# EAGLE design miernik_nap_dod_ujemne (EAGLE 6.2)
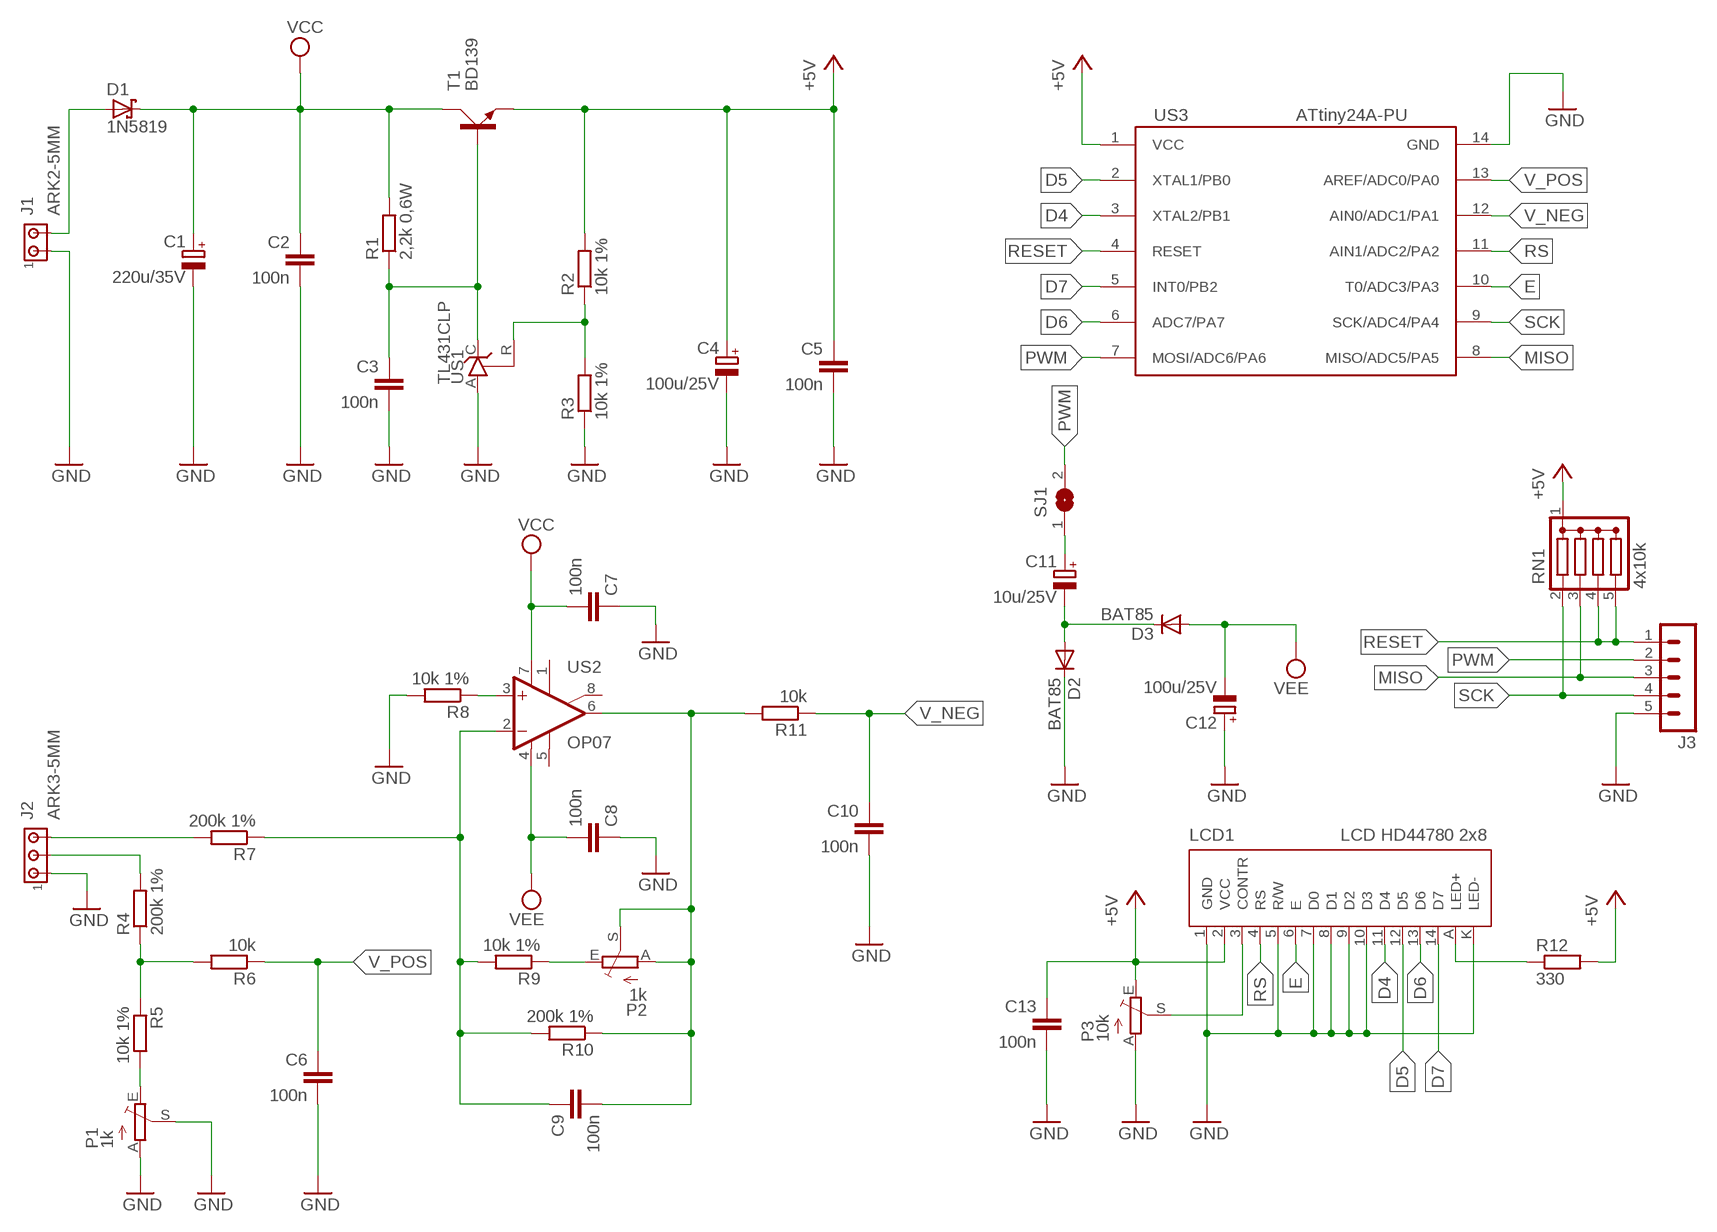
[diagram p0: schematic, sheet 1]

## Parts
C1  220u/35V  CPOL-EUTT5D9L  [TT5D9L]
C2  100n  C-EU050-025X075  [C050-025X075]
C3  100n  C-EU050-030X075  [C050-030X075]
C4  100u/25V  CPOL-EUTT2D6L  [TT2D6L]
C5  100n  C-EU050-025X075  [C050-025X075]
C6  100n  C-EU050-025X075  [C050-025X075]
C7  100n  C-EU050-025X075  [C050-025X075]
C8  100n  C-EU050-025X075  [C050-025X075]
C9  100n  C-EU050-025X075  [C050-025X075]
C10  100n  C-EU050-025X075  [C050-025X075]
C11  10u/25V  CPOL-EUTT2D6L  [TT2D6L]
C12  100u/25V  CPOL-EUTT2D6L  [TT2D6L]
C13  100n  C-EU050-025X075  [C050-025X075]
D1  1N5819  SCHOTTKY-DIODEF126Z12  [F126Z12]
D2  BAT85  BAT81  [DO34-7]
D3  BAT85  BAT81  [DO34-7]
J1  ARK2-5MM  [2PIN-5MM]
J2  ARK3-5MM  [3PIN-5MM]
J3  MA05-1  [MA05-1]
LCD1  LCD HD44780 2x8  LCD_ZLACZE-MINI  [LCD_HD44780_1X6_NAD-ELEMENTAMI_Z-PODSW]
P1  1k  TRIM_EU-B64Y  [B64Y]
P2  1k  TRIM_EU-B64Y  [B64Y]
P3  10k  TRIM_EU-CA6V  [CA6V]
R1  2,2k 0,6W  R-EU_0207/7  [0207/7]
R2  10k 1%  R-EU_0207/7  [0207/7]
R3  10k 1%  R-EU_0207/7  [0207/7]
R4  200k 1%  R-EU_0207/7  [0207/7]
R5  10k 1%  R-EU_0207/7  [0207/7]
R6  10k  R-EU_0207/7  [0207/7]
R7  200k 1%  R-EU_0207/7  [0207/7]
R8  10k 1%  R-EU_0207/7  [0207/7]
R9  10k 1%  R-EU_0207/7  [0207/7]
R10  200k 1%  R-EU_0207/7  [0207/7]
R11  10k  R-EU_0207/7  [0207/7]
R12  330  R-EU_0207/7  [0207/7]
RN1  4x10k  DRAB_REZ_1X4  [RN-5]
SJ1  SJ  [SJ]
T1  BD139  [TO126AV]
US1  TL431CLP  [TO92-CLP]
US2  OP07  OP07N  [DIL08]
US3  ATtiny24A-PU  ATTINY24/44/84-PU  [DIL14]

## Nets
+5V: C4.+ C5.1 C13.1 LCD1.2(VCC) P3.E R2.2 R12.2 RN1.1(C) T1.E US3.1(VCC)
D4: LCD1.11(D4) US3.3(XTAL2/PB1)
D5: LCD1.12(D5) US3.2(XTAL1/PB0)
D6: LCD1.13(D6) US3.6(ADC7/PA7)
D7: LCD1.14(D7) US3.5(INT0/PB2)
E: LCD1.6(E) US3.10(T0/ADC3/PA3)
GND: C1.- C2.2 C3.2 C4.- C5.2 C6.2 C7.1 C8.1 C10.2 C12.+ C13.2 D2.C J1.P$1 J2.P$1 J3.5 LCD1.1(GND) LCD1.5(R/W) LCD1.7(D0) LCD1.8(D1) LCD1.9(D2) LCD1.10(D3) LCD1.K(LED-) P1.A P1.S P3.A R3.1 R8.2 US1.A US3.14(GND)
MISO: J3.3 RN1.3 US3.8(MISO/ADC5/PA5)
N$1: LCD1.3(CONTR) P3.S
N$2: C11.- D2.A D3.C
N$3: C11.+ SJ1.1
N$4: J2.P$2 R4.2
N$5: LCD1.A(LED+) R12.1
N$6: P1.E R5.2
N$7: R4.1 R5.1 R6.2
N$8: D1.A J1.P$2
N$9: R8.1 US2.3(+IN)
N$10: C9.2 P2.A P2.S R10.1 R11.2 US2.6(OUT)
N$11: C3.1 R1.1 T1.B US1.C
N$12: P2.E R9.1
N$14: C9.1 R7.1 R9.2 R10.2 US2.2(-IN)
N$15: J2.P$3 R7.2
N$33: R2.1 R3.2 US1.R
PWM: J3.2 SJ1.2 US3.7(MOSI/ADC6/PA6)
RESET: J3.1 RN1.4 RN1.5 US3.4(RESET)
RS: LCD1.4(RS) US3.11(AIN1/ADC2/PA2)
SCK: J3.4 RN1.2 US3.9(SCK/ADC4/PA4)
V_NEG: C10.1 R11.1 US3.12(AIN0/ADC1/PA1)
V_POS: C6.1 R6.1 US3.13(AREF/ADC0/PA0)
VCC: C1.+ C2.1 C7.2 D1.C R1.2 T1.C US2.7(V+)
VEE: C8.2 C12.- D3.A US2.4(V-)
Unconnected: US2.1(ON1) US2.5(OPT) US2.8(ON2)

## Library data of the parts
C1 C4 C11 C12 = rcl:CPOL-EU: POLARIZED CAPACITOR, European symbol
C2 C3 C5-C10 C13 = rcl:C-EU: CAPACITOR, European symbol
D1 = diode:SCHOTTKY-DIODE: Schottky Diode
D2 D3 = diode:BAT81: DIODE
J1 = zlacza_futrzak:ARK2: ARK 2
J2 = zlacza_futrzak:ARK3: ARK 3 Raster 5mm i 3,5mm
J3 = zlacza_futrzak:MA05-1: PIN HEADER; OC_FARNELL: unknown; OC_NEWARK: unknown
LCD1 = inne_futrzak:LCD_ZLACZE
P1-P3 = pot:TRIM_EU-: POTENTIOMETER
R1-R12 = rcl:R-EU_: RESISTOR, European symbol
RN1 = inne_futrzak:DRAB_REZ_1X4
SJ1 = jumper:SJ: SMD solder JUMPER
T1 = transistor-power:BD139: NPN TRANSISTOR
US1 = v-reg:TL431CLP: VOLTAGE REGULATOR
US2 = linear:OP07*: OP AMP
US3 = scalaki_futrzak:ATTINY24/44/84

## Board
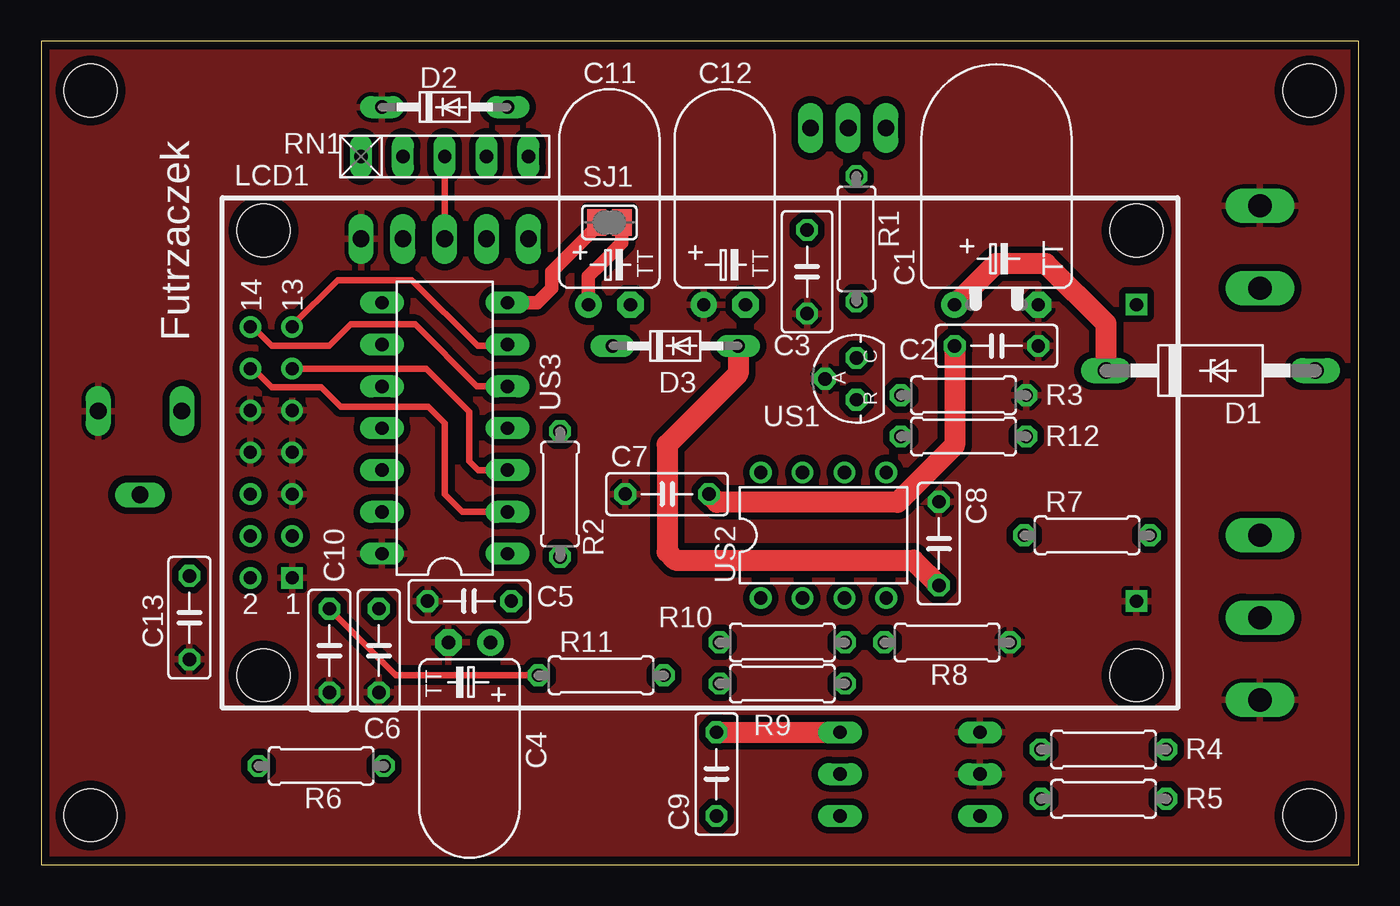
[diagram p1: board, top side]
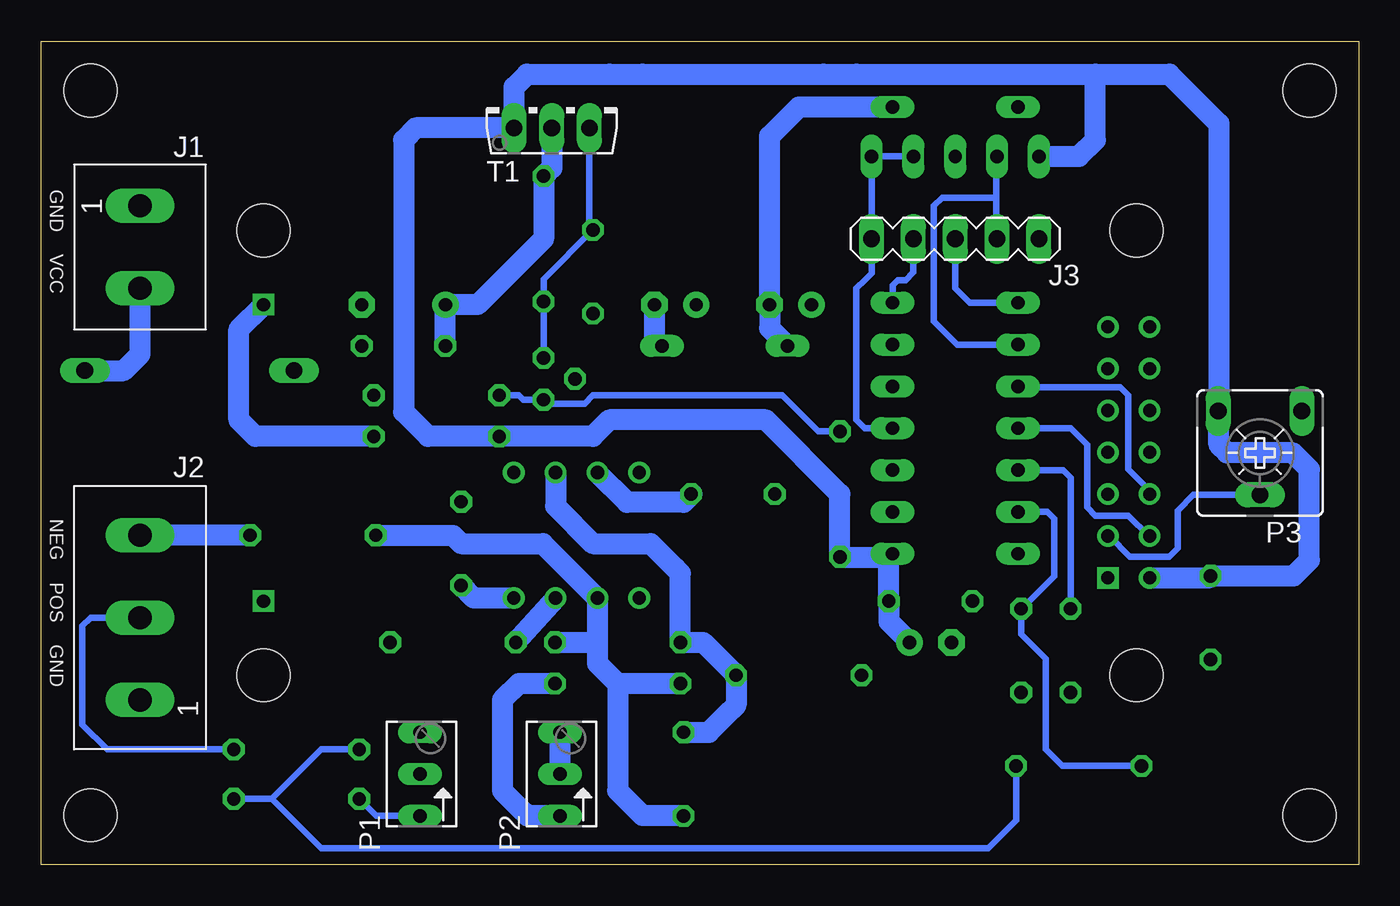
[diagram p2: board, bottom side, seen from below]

Size 80 x 50 mm. Coordinates in mm from the lower left corner, seen from the top.
Outline: 0,0 80,0 80,50 0,50 0,0
Copper layers (1*16): Top 0.035mm / dielectric 1.5mm / Bottom 0.035mm
Design rules: minimum track width 10mil, minimum drill 23mil, track to track 8mil, track to pad 8mil, pad to pad 8mil, via to via 8mil, smd to smd 8mil, copper to edge 20mil, drill to drill 8mil, minimum pad ring 10mil, minimum via ring 8mil, stop-mask expansion 4mil, vias tented up to drill 0mil, thermal gap 10mil
Holes 3.2 mm at 3,3 3,47 77,3 77,47

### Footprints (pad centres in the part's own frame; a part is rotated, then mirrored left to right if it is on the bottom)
TT5D9L = drill 0.813 pad 1.6: + -2.54,0 | drill 0.813 pad 1.6 octagon: - 2.54,0
C050-025X075 = drill 0.813 octagon: 1 -2.54,0; 2 2.54,0
C050-030X075 = drill 0.813 octagon: 1 -2.54,0; 2 2.54,0
TT2D6L = drill 0.813 pad 1.6: + -1.27,0 | drill 0.813 pad 1.6 octagon: - 1.27,0
F126Z12 = drill 1.016 long: A 6.35,0; C -6.35,0
DO34-7 = drill 0.813 long: A 3.81,0; C -3.81,0
2PIN-5MM = drill 1.4 long: P$1 -2.5,0; P$2 2.5,0
3PIN-5MM = drill 1.4 long: P$1 -5,0; P$2 0,0; P$3 5,0
MA05-1 = drill 1.016 long: 1 -5.08,0; 2 -2.54,0; 3 0,0; 4 2.54,0; 5 5.08,0
LCD_HD44780_1X6_NAD-ELEMENTAMI_Z-PODSW = drill 0.8 square: 1 1.74,5.92; A 53,22.5; K 53,4.5 | drill 0.8: 2 -0.8,5.92; 3 1.74,8.46; 4 -0.8,8.46; 5 1.74,11; 6 -0.8,11; 7 1.74,13.54; 8 -0.8,13.54; 9 1.74,16.08; 10 -0.8,16.08; 11 1.74,18.62; 12 -0.8,18.62; 13 1.74,21.16; 14 -0.8,21.16 | hole 3.2: 0,0; 0,27; 53,0; 53,27
B64Y = drill 0.813 long: A 2.54,0; E -2.54,0; S 0,0
CA6V = drill 1.016 long: A -2.54,-2.54; E 2.54,-2.54; S 0,2.54
0207/7 = drill 0.813 octagon: 1 -3.81,0; 2 3.81,0
RN-5 = drill 0.813 long: 1 -5.08,0; 2 -2.54,0; 3 0,0; 4 2.54,0; 5 5.08,0
SJ = smd 1.168 x 1.6: 1 -0.762,0; 2 0.762,0
TO126AV = drill 1.016 long: B 2.286,-1.27; C 0,-1.27; E -2.286,-1.27
TO92-CLP = drill 0.813 octagon: A 0,1.905; C 1.27,0; R -1.27,0
DIL08 = drill 0.813 pad 1.27: 1 -3.81,-3.81; 2 -1.27,-3.81; 3 1.27,-3.81; 4 3.81,-3.81; 5 3.81,3.81; 6 1.27,3.81; 7 -1.27,3.81; 8 -3.81,3.81
DIL14 = drill 0.813 long: 1 -7.62,-3.81; 2 -5.08,-3.81; 3 -2.54,-3.81; 4 0,-3.81; 5 2.54,-3.81; 6 5.08,-3.81; 7 7.62,-3.81; 8 7.62,3.81; 9 5.08,3.81; 10 2.54,3.81; 11 0,3.81; 12 -2.54,3.81; 13 -5.08,3.81; 14 -7.62,3.81

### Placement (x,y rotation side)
C1  58,34 0 top
C2  58,31.5 0 top
C3  46.5,36 270 top
C4  26,13.5 180 top
C5  26,16 180 top
C6  20.5,13 270 top
C7  38,22.5 0 top
C8  54.5,19.5 270 top
C9  41,5.5 90 top
C10  17.5,13 270 top
C11  34.5,34 0 top
C12  41.5,34 0 top
C13  9,15 270 top
D1  71,30 0 top
D2  24.5,46 0 top
D3  38.5,31.5 0 top
J1  74,37.5 270 bottom
J2  74,15 90 bottom
J3  24.5,38 0 bottom
LCD1  13.5,11.5 0 top
P1  57,5.5 90 bottom
P2  48.5,5.5 90 bottom
P3  6,25 180 bottom
R1  49.5,38 90 top
R2  31.5,22.5 270 top
R3  56,28.5 180 top
R4  64.5,7 0 top
R5  64.5,4 180 top
R6  17,6 0 top
R7  63.5,20 0 top
R8  55,13.5 0 top
R9  45,11 180 top
R10  45,13.5 0 top
R11  34,11.5 0 top
R12  56,26 180 top
RN1  24.5,43 0 top
SJ1  34.5,39 180 top
T1  49,46 0 bottom
US1  49.5,29.5 90 top
US2  47.5,20 0 top
US3  24.5,26.5 90 top

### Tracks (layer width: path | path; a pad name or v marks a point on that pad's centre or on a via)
+5V
  Bottom 1.27: LCD1.2 9.12,17.42 C13.1 3.96,17.54 3,18.5 3,24 4,25 8,25 8.5,25.5 8.5,27.5 P3.E 8.5,27.58 8.5,45 11.5,48 16,48 | 16,48 30.5,48 32.5,48 43.5,48 45.5,48 50.5,48 51.29,47.21 T1.E 57.27,44.73 58,44 58,27.5 56.5,26 R12.2 46.5,26 45.5,27 36,27 31.5,22.5 R2.2 31.46,18.65 28.54,18.65 | RN1.1 17,43 16,44 16,48 | 28.54,18.65 C5.1 28.54,14.77 C4.+ | 28.54,18.65 US3.1
D4
  Top 0.406: LCD1.11 23.38,30.12 25,28.5 26,27.5 26,24.5 26.54,23.96 US3.3
D5
  Top 0.406: LCD1.12 12.88,30.12 14,29 17,29 18.2,27.8 23.5,27.8 24.5,26.8 24.5,22.5 25,22 25.58,21.42 US3.2
D6
  Top 0.406: LCD1.13 15.24,32.74 18,35.5 22.5,35.5 26.5,31.5 28.23,31.5 US3.6
D7
  Top 0.406: LCD1.14 12.84,32.66 14,31.5 17.5,31.5 18.8,32.8 22.7,32.8 26.46,29.04 US3.5
E
  Bottom 0.406: LCD1.6 12.7,22.7 14,24 14,28.5 14.5,29 20.65,29 US3.10
GND
  pour Top (isolate 0.406): 0,0 80,0 80,50 0,50
MISO
  Top 0.406: J3.3 RN1.3
  Bottom 0.406: J3.3 24.5,35 23.62,34.12 US3.8
N$1
  Bottom 0.406: LCD1.3 15.16,19.96 13.9,18.7 11.5,18.7 11,19.2 11,21.5 10.04,22.46 P3.S
N$2
  Bottom 1.27: D3.C 35.77,32.58 C11.- 35.77,44.23 35.5,44.5 34,46 D2.A
N$3
  Top 0.813: C11.+ 33.23,35.73 34,36.5 35.26,37.76 SJ1.1
N$4
  Bottom 0.406: J2.P$2 77,15 77.5,14.5 77.5,8.5 76,7 R4.2
N$5
  Bottom 1.27: LCD1.A 68,32.5 68,27 67,26 R12.1
N$6
  Bottom 0.406: P1.E 59.65,2.96 R5.2
N$7
  Bottom 0.406: R5.1 66,4 | 66,4 63,7 R4.1 | 66,4 63,1 53.5,1 22.5,1 21.5,2 20.81,2.69 R6.2
N$8
  Bottom 1.27: D1.A 75,30 74,31 J1.P$2
N$9
  Bottom 1.27: R8.1 US2.3
N$10
  Top 1.27: C9.2 P2.A
  Bottom 1.27: P2.S P2.A | C9.2 39.46,8.04 38.5,9 37.81,9.69 R11.2 39.81,13.5 R10.1 41.19,17.69 41.5,18 43,19.5 46.5,19.5 48.77,21.77 US2.6
N$11
  Bottom 0.406: US1.C R1.1 49.5,35.54 C3.1 46.71,38.75 T1.B
N$12
  Bottom 1.27: R9.1 51,11 52,10 52,4.5 51,3.5 50.46,2.96 P2.E
N$14
  Bottom 1.27: 46.23,13.5 US2.2 49.54,19.5 54.5,19.5 55,20 R7.1 | 46.23,13.5 46.23,12.23 45,11 | 45,11 45,4.5 43.5,3 41.04,3 C9.1 | R9.2 45,11 | R10.2 46.23,13.5
N$15
  Bottom 1.27: R7.2 J2.P$3
N$33
  Bottom 0.406: R3.2 51,28.5 50.73,28.23 US1.R 49.27,28 47,28 46.5,28.5 35,28.5 32.81,26.31 R2.1
PWM
  Top 0.813: SJ1.2 33.74,38.74 31,36 31,35 30.5,34.5 30.12,34.12 US3.7
  Bottom 0.406: US3.7 28.31,35.19 28,35.5 27.5,35.5 27.04,35.96 J3.2
RESET
  Bottom 0.406: US3.4 30,26.5 30.5,27 30.5,32.5 30.5,35 30,35.5 29.58,35.92 J3.1 RN1.5 RN1.4
RS
  Bottom 0.406: LCD1.4 12.76,19.96 14,21.2 16,21.2 16.5,21.7 16.5,25.5 17.5,26.5 US3.11
SCK
  Bottom 0.406: J3.4 22,38.04 22,40 22,40.5 | 22,40.5 22,42.96 RN1.2 | 22,40.5 22.5,40.5 25.3,40.5 25.8,40 25.8,33 24.38,31.58 US3.9
V_NEG
  Top 0.406: R11.1 21.54,11.5 C10.1
  Bottom 0.406: US3.12 17.96,23.96 17.5,23.5 17.5,19.5 17.5,19 C10.1
V_POS
  Bottom 0.406: US3.13 18.92,21.42 18.5,21 18.5,20.5 18.5,17.5 20.46,15.54 C6.1 20.5,14 19,12.5 19,7 18,6 R6.1
VCC
  Top 1.27: D1.C 64.65,32.85 61,36.5 57.96,36.5 C1.+ | C2.1 55.46,25.46 52,22 41.04,22 C7.2
  Bottom 1.27: T1.C 49,42.31 R1.2 49.5,38 53.5,34 C1.+ C2.1 | C7.2 40.5,22.5 41,22 44.42,22 US2.7
VEE
  Top 1.27: D3.A 42.31,29.81 38,25.5 38,19 38.5,18.5 52.96,18.5 C8.2
  Bottom 1.27: C12.- 42.77,31.96 D3.A | US2.4 53.73,16.19 C8.2

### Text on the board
tPlace: Futrzaczek
bPlace: GND VCC | NEG POS GND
